FUNCTION FC 12 : VOID
TITLE =
VERSION : 0.1


VAR_INPUT
  Groesse : INT ;
  LI1 : BOOL ;
  Zeitglied : TIMER ;
  Zeitw_1 : S5TIME ;
  Zeitw_2 : S5TIME ;
  Zeitw_3 : S5TIME ;
  Zeitw_4 : S5TIME ;
END_VAR
VAR_OUTPUT
  Y : BOOL ;
END_VAR
VAR_TEMP
  Zeit : S5TIME ;
END_VAR
BEGIN
NETWORK
TITLE =
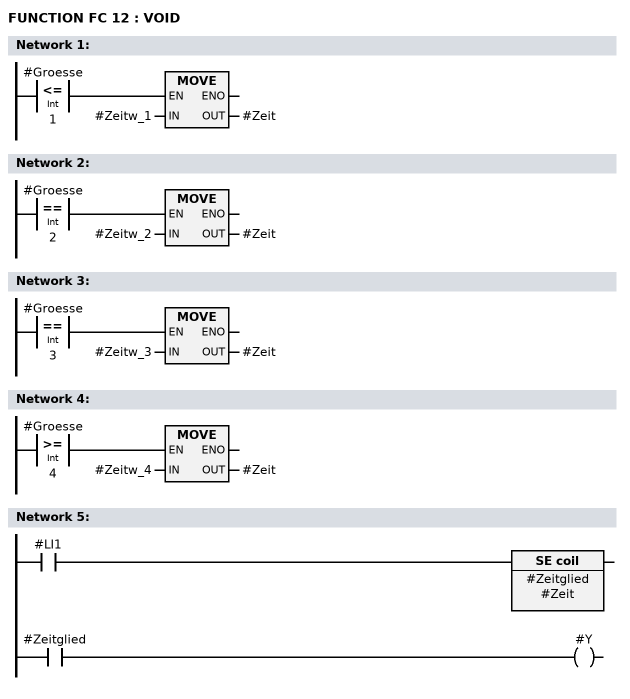
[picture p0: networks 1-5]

      U(    ;
      L     #Groesse;
      L     1;
      <=I   ;
      )     ;
      SPBNB _001;
      L     #Zeitw_1;
      T     #Zeit;
_001: NOP   0;
NETWORK
TITLE =

      U(    ;
      L     #Groesse;
      L     2;
      ==I   ;
      )     ;
      SPBNB _002;
      L     #Zeitw_2;
      T     #Zeit;
_002: NOP   0;
NETWORK
TITLE =

      U(    ;
      L     #Groesse;
      L     3;
      ==I   ;
      )     ;
      SPBNB _003;
      L     #Zeitw_3;
      T     #Zeit;
_003: NOP   0;
NETWORK
TITLE =

      U(    ;
      L     #Groesse;
      L     4;
      >=I   ;
      )     ;
      SPBNB _004;
      L     #Zeitw_4;
      T     #Zeit;
_004: NOP   0;
NETWORK
TITLE =

      U     #LI1;
      L     #Zeit;
      SV    #Zeitglied;
      NOP   0;
      NOP   0;
      NOP   0;
      U     #Zeitglied;
      =     #Y;
END_FUNCTION

